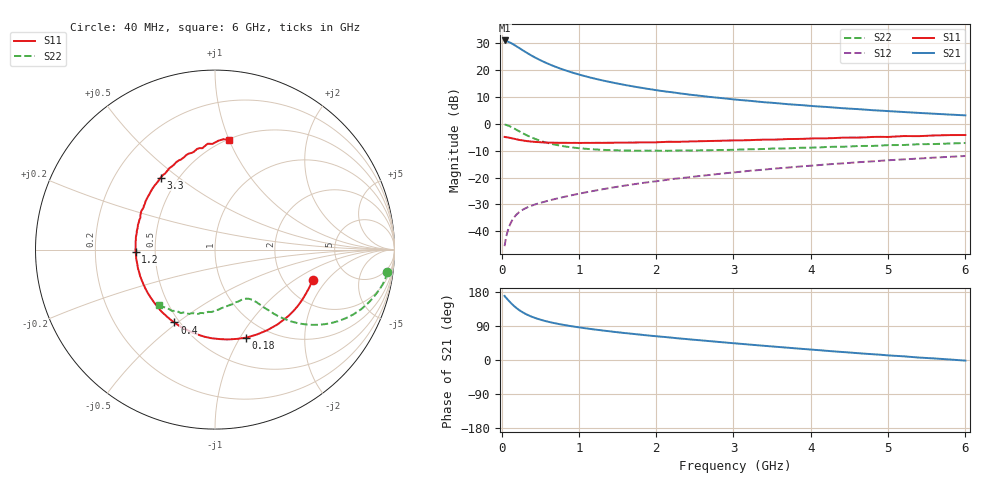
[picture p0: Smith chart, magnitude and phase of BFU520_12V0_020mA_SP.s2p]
! Filename:  P:\Prog\Test\Noise\ATS_data\Testdata_Net\03 Spar\BFU520_APG2013_37_A05_12p0V_020mA_SP_CM01_D.s2p
! Date/Time: Fri 26/Apr/2013 13:00:12
! BFU520_APG2013_37_A05_12p0V_1to20mA_SP_CM01_Bias8_R.s2p
! MDIF S-parameter v. bias file
! BFU520_APG2013_37_A05_12p0V_1to20mA_SP_CM01
! Date/time Tue Apr 23 18:22:57 2013
! VAR V_out= 12.0000
! VAR I_out= 19.9950
! VAR V_in= 0.7897
! VAR I_in= 0.2066
! Device data file deembeded for feedlines and parallel
! Original file: \03 Spar\BFU520_APG2013_37_A05_12p0V_020mA_SP_CM01_R.s2p
! Feed-files: PR047V01_250413_Feed1.s2p, PR047V01_250413_Feed2.s2p
! Parallel-file: PR047V01_250413_Par.s2p
# MHz S MA R 50
!  Freq-MHz  S11-mag  S11-arg  S21-mag  S21-arg  S12-mag  S12-arg  S22-mag  S22-arg
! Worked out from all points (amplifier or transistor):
!   98 points, 40 MHz to 6 GHz, reference 50 ohm
!   highest |S21| = 31.0 dB at 40 MHz (marker M1)
!   |S21| within 3 dB of that: start of sweep to 239 MHz
!   unconditionally stable (mu >= 1): 1.466 GHz to 3.503 GHz
!   at 300 MHz: K = 0.44, MSG = 29.2 dB, |S12| = -31.5 dB
!   at 1.6 GHz: K = 1.02, MAG = 17.9 dB, |S12| = -23.0 dB
!   at 6 GHz: K = 0.85, MSG = 7.6 dB, |S12| = -12.0 dB
!   S11 on the Smith chart (normalised r, x): 40 MHz: 2.86, -1.43; 180 MHz: 0.79, -1.06; 400 MHz: 0.47, -0.49; 1.2 GHz: 0.39, -0.01; 3.3 GHz: 0.40, +0.43; 6 GHz: 0.50, +1.00
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40  0.5698 -17.2  35.4 169.1  0.005309 81.8  0.9676 -7.5
50  0.5664 -21.7  35.35 166.0  0.006598 80.2  0.9632 -9.6
90  0.5549 -38.2  33.3 157.2  0.01129 74.3  0.9196 -17.1
120  0.5435 -50.0  31.86 150.6  0.01443 70.2  0.88 -22.1
140  0.5353 -57.1  30.69 146.6  0.01628 67.8  0.8509 -25.1
180  0.5205 -70.5  28.34 139.4  0.01959 63.9  0.7932 -30.2
220  0.5055 -82.1  26.12 133.0  0.02227 60.9  0.737 -34.4
280  0.4889 -97.0  22.98 125.2  0.02553 57.7  0.6615 -39.1
340  0.4738 -109.1  20.36 118.8  0.02817 55.7  0.5997 -42.5
400  0.4648 -119.1  18.15 113.5  0.03042 54.7  0.5485 -44.8
500  0.4546 -132.5  15.26 106.7  0.03389 54.1  0.4849 -47.5
650  0.4458 -147.2  12.23 98.8  0.03869 54.6  0.4219 -49.8
800  0.4425 -157.8  10.15 92.8  0.04345 55.8  0.3832 -51.3
1050  0.441 -171.7  7.884 84.7  0.05174 57.5  0.347 -53.8
1200  0.4422 -178.1  6.941 80.6  0.05688 58.3  0.3343 -55.3
1600  0.4463 167.6  5.256 71.0  0.07111 59.2  0.3187 -60.4
2050  0.4564 155.8  4.115 61.8  0.08722 59.1  0.3158 -67.5
3100  0.4929 131.0  2.758 42.6  0.1287 56.0  0.3325 -85.4
3300  0.5026 127.0  2.596 39.1  0.1371 54.9  0.337 -88.8
4100  0.5363 111.9  2.097 26.0  0.1704 50.0  0.3627 -103.0
5200  0.5914 94.0  1.656 9.7  0.218 41.9  0.403 -122.1
6000  0.6178 82.8  1.435 -1.6  0.2519 35.1  0.44 -135.6
